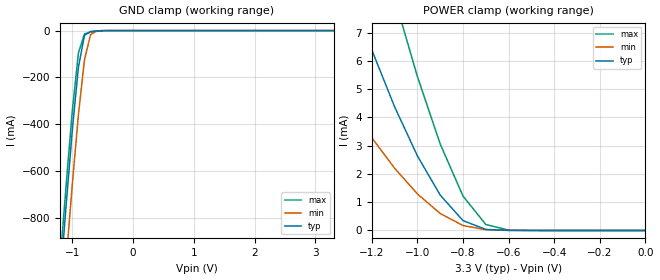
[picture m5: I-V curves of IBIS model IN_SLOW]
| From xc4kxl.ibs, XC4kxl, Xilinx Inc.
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|   Model IN_SLOW
[Model]   IN_SLOW
Model_type   Input
Polarity   Non-Inverting
Vinl = 0.800V
Vinh = 2.000V
C_comp   7.0000pF   6.0000pF   8.0000pF
[Temperature Range]   27.0000   100.0000   0.000
[Voltage Range]   3.3000V   3.0000V   3.6000V
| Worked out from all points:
|   GND clamp passes 1 mA (typ) near -0.58 V on its own axis
|   POWER clamp passes 1 mA (typ) near -0.87 V on its own axis
[GND_clamp]
| voltage   I(typ)   I(min)   I(max)
-3.3V     -8.626A    -8.837A    -8.551A
-1.2V     -1.073A    -1.312A    -987.3mA
-1.1V     -740.8mA   -978.2mA   -654.8mA
-1V       -426mA     -657.1mA   -343.9mA
-900mV    -157.2mA   -360.9mA   -96.62mA
-800mV    -20.77mA   -124.4mA   -14.17mA
-700mV    -3.846mA   -17.61mA   -6.82mA
-600mV    -1.246mA   -1.662mA   -3.283mA
-300mV    -276.3nA   -435.5nA   -2.755uA
3.3V      151.6pA    7.389nA    160.2pA
[POWER_clamp]
| voltage   I(typ)   I(min)   I(max)
-3.3V     75.42mA    47.28mA    100.2mA
-1.5V     13.67mA    7.363mA    21.72mA
-1.4V     11.06mA    5.873mA    18.06mA
-1.3V     8.626mA    4.508mA    14.56mA
-1.2V     6.385mA    3.279mA    11.27mA
-1.1V     4.373mA    2.199mA    8.21mA
-1V       2.636mA    1.293mA    5.443mA
-900mV    1.25mA     599.1uA    3.055mA
-800mV    347.4uA    174.4uA    1.214mA
-700mV    37.68uA    27.06uA    209.3uA
-600mV    2.828uA    3.397uA    13.73uA
0V        151.6pA    186.1pA    177.1pA
